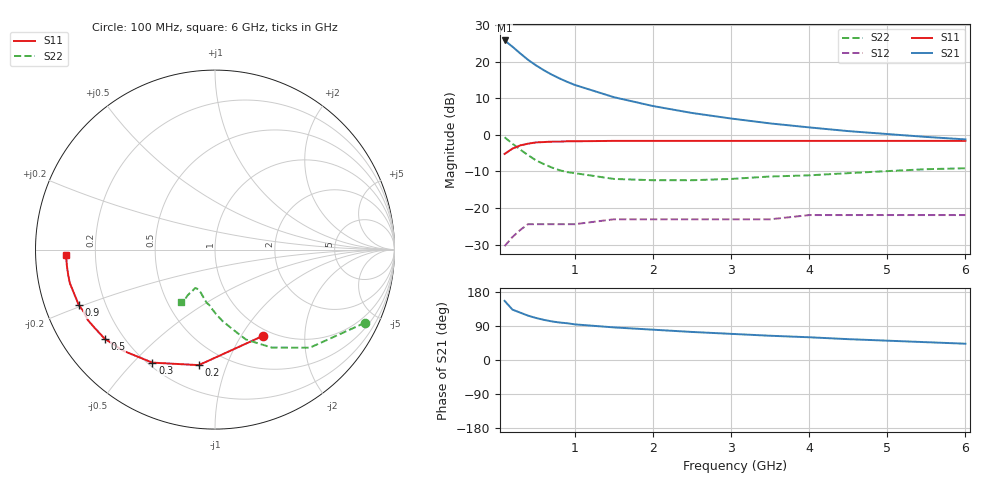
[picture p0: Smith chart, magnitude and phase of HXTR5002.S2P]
! HXTR-5002 Common Emitter
! Vce=18V Ic=110ma
# ghz s ma r 50
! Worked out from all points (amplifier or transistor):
!   20 points, 100 MHz to 6 GHz, reference 50 ohm
!   highest |S21| = 25.9 dB at 100 MHz (marker M1)
!   |S21| within 3 dB of that: start of sweep to 270.5 MHz
!   unconditionally stable (mu >= 1): 2.71 GHz to end of sweep
!   at 400 MHz: K = 0.16, MSG = 22.5 dB, |S12| = -24.4 dB
!   at 1.5 GHz: K = 0.55, MSG = 16.7 dB, |S12| = -23.1 dB
!   at 6 GHz: K = 1.71, MAG = 5.5 dB, |S12| = -21.9 dB
!   S11 on the Smith chart (normalised r, x): 100 MHz: 0.91, -1.25; 200 MHz: 0.36, -0.80; 300 MHz: 0.22, -0.57; 500 MHz: 0.13, -0.35; 900 MHz: 0.10, -0.19; 6 GHz: 0.09, -0.02
0.1  0.55 -61.0  19.7 156.0  0.03 68.0  0.93 -26.0
0.2  0.65 -98.0  16.2 133.0  0.04 50.0  0.76 -46.0
0.3  0.72 -119.0  13.1 125.0  0.05 39.0  0.63 -60.0
0.4  0.76 -132.0  10.7 117.0  0.06 32.0  0.53 -71.0
0.5  0.79 -141.0  9.01 111.0  0.06 27.0  0.45 -78.0
0.6  0.8 -147.0  7.73 106.0  0.06 24.0  0.4 -84.0
0.7  0.81 -151.0  6.74 102.0  0.06 22.0  0.36 -89.0
0.8  0.81 -155.0  5.97 99.0  0.06 20.0  0.33 -93.0
0.9  0.82 -158.0  5.35 97.0  0.06 19.0  0.31 -96.0
1  0.82 -160.0  4.84 94.0  0.06 18.0  0.3 -99.0
1.5  0.83 -167.0  3.29 86.0  0.07 16.0  0.25 -109.0
2  0.83 -170.0  2.49 80.0  0.07 16.0  0.24 -114.0
2.5  0.83 -173.0  2 74.0  0.07 17.0  0.24 -117.0
3  0.83 -174.0  1.68 69.0  0.07 18.0  0.25 -118.0
3.5  0.83 -175.0  1.44 64.0  0.07 19.0  0.27 -119.0
4  0.83 -176.0  1.27 60.0  0.08 20.0  0.28 -120.0
4.5  0.83 -177.0  1.13 55.0  0.08 21.0  0.3 -121.0
5  0.83 -177.0  1.03 51.0  0.08 21.0  0.32 -121.0
5.5  0.83 -178.0  0.94 47.0  0.08 22.0  0.34 -122.0
6  0.83 -178.0  0.87 43.0  0.08 22.0  0.35 -123.0
